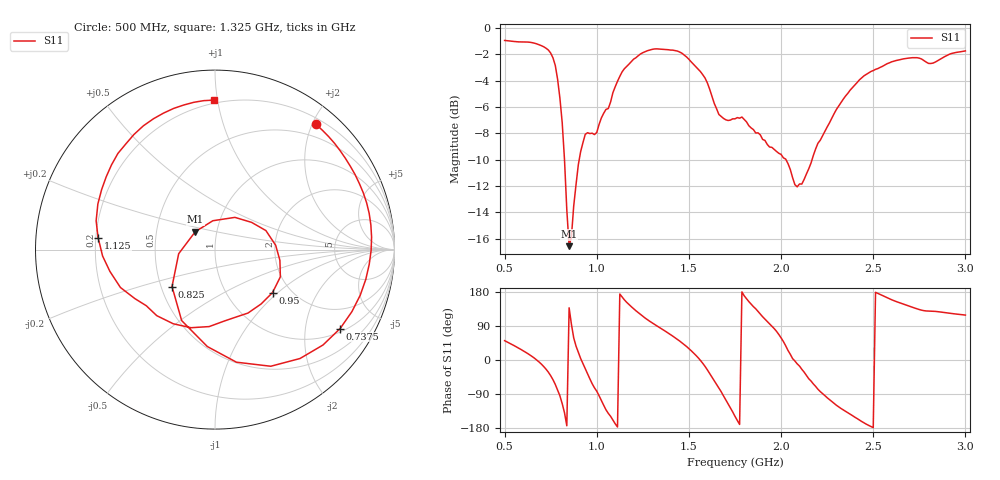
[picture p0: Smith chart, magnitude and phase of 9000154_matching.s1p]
#  HZ  S  DB  R  50.00
! Rohde & Schwarz Vector Network Analyzer
! Rohde-Schwarz,ZNB8-4Port,1311601044101844,3.45
! Created: UTC 10/4/2024, 7:18:26 AM
! freq[Hz]  db:S22  ang:S22
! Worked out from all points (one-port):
!   201 points, 500 MHz to 3 GHz, reference 50 ohm
!   lowest |S11| = -16.6 dB at 850 MHz (marker M1), VSWR 1.35, Z = 39.4 + j8.04 ohm
!   |S11| at or under -10 dB: 824.9 MHz to 904.8 MHz (79.88 MHz wide, 9.24 % of centre); 2.026 GHz to 2.168 GHz (141.7 MHz wide, 6.76 % of centre)
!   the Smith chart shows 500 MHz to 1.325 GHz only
!   S11 on the Smith chart (normalised r, x): 500 MHz: 0.29, +2.06; 737.5 MHz: 1.12, -3.08; 825 MHz: 0.57, -0.26; 950 MHz: 1.62, -0.92; 1.125 GHz: 0.21, +0.05; 1.325 GHz: 0.18, +0.98
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5e8  -0.95 51.0
6.5e8  -1.12 9.0
7.375e8  -1.68 -32.2
7.75e8  -2.85 -64.5
8.125e8  -7.19 -115.2
8.25e8  -10.01 -139.3
8.5e8  -16.57 137.7
8.875e8  -11.90 36.7
9.5e8  -7.96 -36.8
1.025e9  -6.83 -107.1
1.125e9  -3.68 174.1
1.2375e9  -1.97 120.0
1.325e9  -1.59 90.4
1.4375e9  -1.75 54.4
1.5125e9  -2.58 24.5
1.575e9  -3.55 -8.7
1.65e9  -6.13 -63.8
1.7e9  -6.97 -104.9
1.75e9  -6.90 -148.7
1.7875e9  -6.77 179.7
1.8875e9  -8.12 120.7
1.9875e9  -9.52 67.5
2.0625e9  -11.37 3.7
2.2375e9  -7.84 -93.9
2.375e9  -4.72 -143.0
2.5125e9  -3.14 178.6
2.6875e9  -2.30 143.5
3e9  -1.74 118.5
